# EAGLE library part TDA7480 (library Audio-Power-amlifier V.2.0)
The TDA7480 is an audio class-D amplifier assembled in Power DIP package specially designed for high efficiency applications mainly for TV and Home Stereo sets.
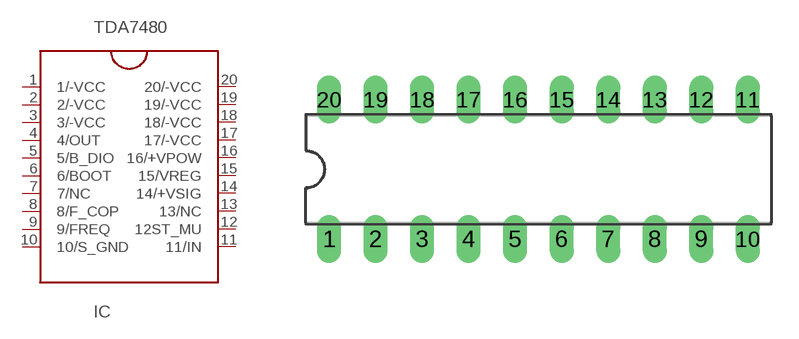
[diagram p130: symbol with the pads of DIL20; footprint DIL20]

Designator prefix IC

## TDA7480  [DIL20]
1  1/-VCC  pwr
2  2/-VCC  pwr
3  3/-VCC  pwr
4  4/OUT  out
5  5/B_DIO
6  6/BOOT
7  7/NC  nc
8  8/F_COP
9  9/FREQ
10  10/S_GND  pwr
11  11/IN  in
12  12ST_MU  in
13  13/NC  nc
14  14/+VSIG  pwr
15  15/VREG
16  16/+VPOW  pwr
17  17/-VCC  pwr
18  18/-VCC  pwr
19  19/-VCC  pwr
20  20/-VCC  pwr

## Footprint DIL20 (pad centres in mm)
Dual In Line Package
drill 0.813 long: 1 -11.43,-3.81; 2 -8.89,-3.81; 3 -6.35,-3.81; 4 -3.81,-3.81; 5 -1.27,-3.81; 6 1.27,-3.81; 7 3.81,-3.81; 8 6.35,-3.81; 9 8.89,-3.81; 10 11.43,-3.81; 11 11.43,3.81; 12 8.89,3.81; 13 6.35,3.81; 14 3.81,3.81; 15 1.27,3.81; 16 -1.27,3.81; 17 -3.81,3.81; 18 -6.35,3.81; 19 -8.89,3.81; 20 -11.43,3.81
